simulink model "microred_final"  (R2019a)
settings: Solver=VariableStepAuto  StartTime=0.0  StopTime=24*60*60  FixedStep=1  RelTol=1e-3
undefined symbols (not defined in the file): A, B, C, cargagenerador, CoeficienteProduccion, Consumo_valores, consumogenerador, D1, Dd, Delta, irradiancia_valores, j, magnitude, PotenciaAerogenerador, precioelectricidad_valores, Precioventaelectricidad, Tiempo, VelocidadAerogenerador, viento_valores
libraries: powerlib x42, powerlib_meascontrol x6
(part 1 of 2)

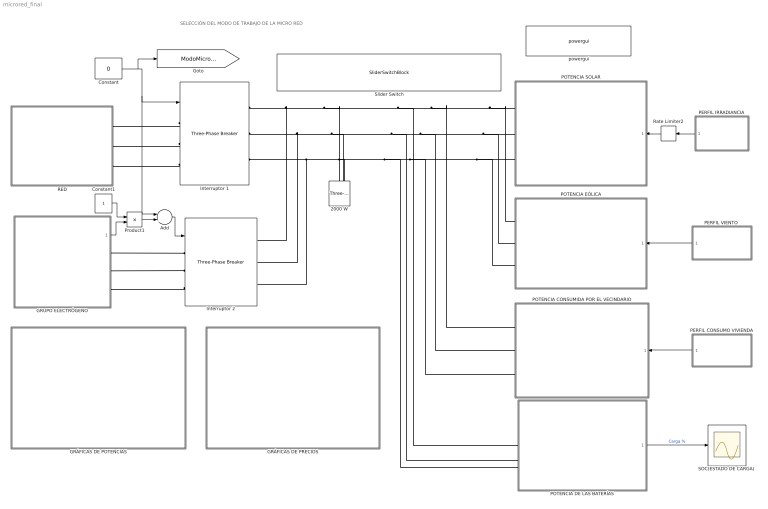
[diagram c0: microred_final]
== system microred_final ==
  note: SELECCIÓN DEL MODO DE TRABAJO DE LA MICRO RED
  2000 W : powerlib/Elements/Three-Phase Series RLC Load  LConnTagsString=A|B|C  Configuration=Y (grounded)  NominalVoltage=25e3  Vabc=[1e3 1e3 1e3]  Vabcp=[1e3 1e3 1e3]  NominalFrequency=50  UnbalancedPower=off  ActivePower=2000  InductivePower=0  CapacitivePower=0  Pabc=[10e3 9e3 11e3]  QLabc=[100 90 110]  QCabc=[100 90 110]  Pabcp=[10e3 9e3 11e3]  QLabcp=[100 90 110]  QCabcp=[100 90 110]  Measurements=None  LoadType=constant Z
  Add : Sum  Inputs=-+
  Constant : Constant  Value=0
  Constant1 : Constant
  GRUPO ELECTRÓGENO : Subsystem  mask{Voltaje=380, PotenciaMax=400}
      mask prompts: Voltaje "Voltaje (v)"; PotenciaMax "Potencia máxima (KW)"
  GRÁFICAS DE POTENCIAS : Subsystem
  GRÁFICAS DE PRECIOS : Subsystem
  Interruptor 1 : powerlib/Elements/Three-Phase Breaker  InitialState=closed  SwitchA=on  SwitchB=on  SwitchC=on  SwitchTimes="[1/60  5/60]"  External=on  BreakerResistance=0.001  SnubberResistance=100e6  SnubberCapacitance=0  Measurements=None
  Interruptor 2 : powerlib/Elements/Three-Phase Breaker  InitialState=closed  SwitchA=on  SwitchB=on  SwitchC=on  SwitchTimes="[1/60  5/60]"  External=on  BreakerResistance=0.001  SnubberResistance=inf  SnubberCapacitance=0  Measurements=None
  PERFIL CONSUMO VIVIENDA : Subsystem
      mask init:
      | load microred
  PERFIL IRRADIANCIA : Subsystem
      mask init:
      | load microred
  "PERFIL VIENTO " : Subsystem
      mask init:
      | load microred
  POTENCIA CONSUMIDA POR EL VECINDARIO : Subsystem  mask{NumCasas=1200, Fdp=0.8}
      mask prompts: NumCasas "Número de Casas"; Fdp "Factor de Potencia(0.8-1)"
  POTENCIA DE LAS BATERÍAS : Subsystem  mask{Rendimiento=95, Capacidad=4600, Vbat=400, Pbat=9200, NumBat=200, L_Sup=85, L_Inf=15, EstadoInicial=49.400, ModoEnergetico=Optimización de la energia}
      mask prompts: Rendimiento "Rendimiento de las baterías(%)"; Capacidad "Capacidad de las baterías(Ah)"; Vbat "Tensión de las baterías"; Pbat "Potencia de cada batería"; NumBat "Número de baterías"; L_Sup "Limite supeior SOC baterías"; L_Inf "Limite infeior SOC baterías"; EstadoInicial "Estado Inicial De la Carga(%)"; ModoEnergetico "Modo concetado a red"
  POTENCIA EÓLICA : Subsystem  mask{Modo=Curva de potencia, Densidad=1.225, SupViento=75.4, NumAerogeneradores=20, Fp=0.95}
      mask prompts: Modo "Modo de trabajo"; Densidad "Densidad del viento (kg/m^3)"; SupViento "Superficie de viento que incide en las aspas (m2)"; NumAerogeneradores "Número de aerogeneradores"; Fp "Factor de potencia ( 0.9-1)"
  POTENCIA SOLAR : Subsystem  mask{AreaPanel=1.77, NumPaneles=600, RendimientoPanel=22.6, Fdp=0.95}
      mask prompts: AreaPanel "Área de Cada Panel Solar (m^2)"; NumPaneles "Número de Paneles Solares"; RendimientoPanel "Rendimiento de los paneles solares (%)"; Fdp "Factor de Potencia (0.9-1)"
  Product1 : Product
  RED : Subsystem
  Rate Limiter2 : RateLimiter  RisingSlewLimit=1e7  FallingSlewLimit=-1e7  SampleTimeMode=inherited
  "SOC(ESTADO DE CARGA) " : Scope
  Slider Switch : SliderSwitchBlock
  powergui : powerlib/powergui  Priority=1  SimulationMode=Phasor  SampleTime=50e-6  frequency=50  Iterations=50  frequencyindice=50  Pbase=100e6  ErrMax=1e-4  UnitsV=kV  UnitsW=MW  buscounter=0  FunctionMessages=off  echomessages=off  EnableUseOfTLC=off  CurrentSourceSwitches=off  DisableSnubberDevices=off  DisableRonSwitches=off  DisableVfSwitches=off  DisplayEquations=off  AutomaticDiscreteSolvers=off  SolverType=Tustin/Backward Euler (TBE)  Interpol=off  ExternalGateDelay=off  methode=off  Ts=100  x0status=blocks  SPID=on  SwTol=0  HookPort=off  NonlinearTolerance=0  nMaxIteration=15  ContinueOnMaxIteration=off  RestoreLinks=warning  ResistiveCurrentMeasurement=off  Frange=[0:2:500]  Ylog=off  Xlog=on  ShowGrid=off  save=off  variable=ZData  structure=0  ZoomFFT=off  StartTime=0.0  cycles=1  DisplayStyle=1  fundamental=60  FreqAxis=off  MaxFrequency=1000  frequencyindicesteady=1  RmsSteady=1  display=off
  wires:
  POTENCIA DE LAS BATERÍAS/1(SOC) -> "SOC(ESTADO DE CARGA) "/1  "Carga %"
  Constant1/1 -> Product1/1
  GRUPO ELECTRÓGENO/1(Valor Coparacion Potencias) -> Product1/2
  Add/1 -> Interruptor 2/1
  Product1/1 -> Add/2
  Rate Limiter2/1 -> POTENCIA SOLAR/1(Perfil irradiancia)
  PERFIL CONSUMO VIVIENDA/1(Out2) -> POTENCIA CONSUMIDA POR EL VECINDARIO/1("Perfil consumo vivienda ")
  "PERFIL VIENTO "/1(Out2) -> POTENCIA EÓLICA/1(Perfil de viento)
  PERFIL IRRADIANCIA/1(Out1) -> Rate Limiter2/1
  Constant/1 -> [ModoMicrorred], Add/1, Interruptor 1/1
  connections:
  Interruptor 1/RConn2 -- Interruptor 2/RConn2 -- POTENCIA EÓLICA/RConn2 -- POTENCIA SOLAR/RConn2 -- POTENCIA CONSUMIDA POR EL VECINDARIO/RConn2 -- POTENCIA DE LAS BATERÍAS/LConn2 -- 2000 W/LConn2
  Interruptor 1/RConn3 -- Interruptor 2/RConn3 -- POTENCIA CONSUMIDA POR EL VECINDARIO/RConn3 -- POTENCIA EÓLICA/RConn3 -- POTENCIA SOLAR/RConn3 -- POTENCIA DE LAS BATERÍAS/LConn3 -- 2000 W/LConn3
  Interruptor 1/RConn1 -- Interruptor 2/RConn1 -- POTENCIA SOLAR/RConn1 -- POTENCIA EÓLICA/RConn1 -- POTENCIA CONSUMIDA POR EL VECINDARIO/RConn1 -- POTENCIA DE LAS BATERÍAS/LConn1 -- 2000 W/LConn1
  Interruptor 2/LConn3 -- GRUPO ELECTRÓGENO/RConn3
  Interruptor 2/LConn1 -- GRUPO ELECTRÓGENO/RConn1
  Interruptor 1/LConn3 -- RED/RConn3
  Interruptor 2/LConn2 -- GRUPO ELECTRÓGENO/RConn2
  Interruptor 1/LConn2 -- RED/RConn2
  Interruptor 1/LConn1 -- RED/RConn1

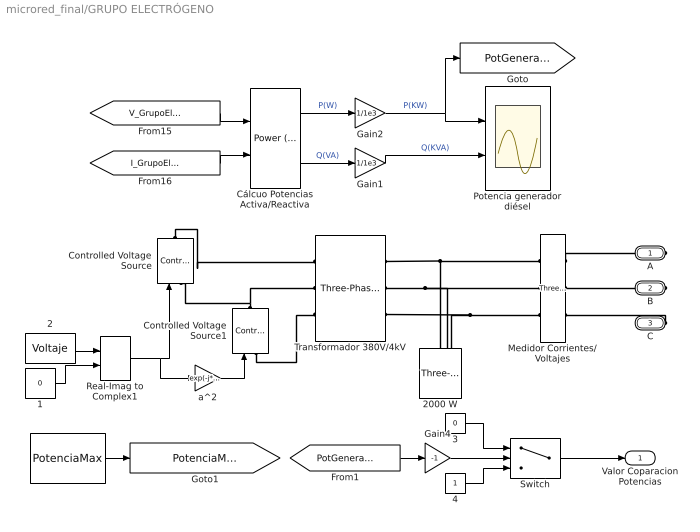
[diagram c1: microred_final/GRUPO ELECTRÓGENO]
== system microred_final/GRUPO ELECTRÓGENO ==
  " " : Constant  Value=PotenciaMax
  1 : Constant  Value=0
  2 : Constant  Value=Voltaje
  2000 W : powerlib/Elements/Three-Phase Series RLC Load  LConnTagsString=A|B|C  Configuration=Y (grounded)  NominalVoltage=25e3  Vabc=[1e3 1e3 1e3]  Vabcp=[1e3 1e3 1e3]  NominalFrequency=50  UnbalancedPower=off  ActivePower=2000  InductivePower=0  CapacitivePower=0  Pabc=[10e3 9e3 11e3]  QLabc=[100 90 110]  QCabc=[100 90 110]  Pabcp=[10e3 9e3 11e3]  QLabcp=[100 90 110]  QCabcp=[100 90 110]  Measurements=None  LoadType=constant Z
  3 : Constant  Value=0
  4 : Constant
  Controlled Voltage Source : powerlib/Electrical Sources/Controlled Voltage Source  Initialize=on  Source_Type=AC  Amplitude=0  Phase=0  Frequency=50  Measurements=None
  Controlled Voltage Source1 : powerlib/Electrical Sources/Controlled Voltage Source  Initialize=on  Source_Type=AC  Amplitude=0  Phase=0  Frequency=50  Measurements=None
  Cálcuo Potencias Activa/Reactiva : powerlib_meascontrol/Measurements/Power (3ph, Phasor)
  Gain1 : Gain  Gain=1/1e3
  Gain2 : Gain  Gain=1/1e3
  Gain4 : Gain  Gain=-1
  Medidor Corrientes/Voltajes : powerlib/Measurements/Three-Phase V-I Measurement  VoltageMeasurement=phase-to-ground  SetLabelV=on  LabelV=V_GrupoElectrogeno  Vpu=off  VpuLL=off  CurrentMeasurement=yes  SetLabelI=on  LabelI=I_GrupoElectrogeno  Ipu=off  Pbase=2*1.5e6/0.9  Vbase=25e3  OutputType=Complex  PhasorSimulation=on  PSBequivalent=0
  Potencia generador diésel : Scope  NumInputPorts=2
  Real-Imag to Complex1 : RealImagToComplex
  Switch : Switch  Criteria=u2 > Threshold  Threshold=PotenciaMax
  Transformador 380V/4kV : powerlib/Elements/Three-Phase Transformer (Two Windings)  Winding1Connection=Delta (D1)  Winding2Connection=Yg  CoreType=Three single-phase transformers  SetSaturation=off  Hysteresis=off  DataFile='hysteresis'  SetInitialFlux=off  Measurements=None  UNITS=pu  NominalPower=[ 20e6 , 60 ]  Winding1=[Voltaje, 0.002 , 0.08 ]  Winding2=[ 4000 , 0.002 , 0.08 ]  Rm=500  Lm=500  L0=0.5  Saturation=[ 0,0 ; 0.0024,1.2 ; 1.0,1.52 ]  InitialFluxes=[ 0.8 , -0.8 , 0.7 ]  BreakLoop=off  DiscreteSolver=Trapezoidal iterative  DataType=off  TransfoNumber=1
  a^2 : Gain  Gain=exp(-j*2*pi/3)
  A : PMIOPort  Side=Right
  B : PMIOPort  Port=2  Side=Right
  C : PMIOPort  Port=3  Side=Right
  Valor Coparacion Potencias : Outport
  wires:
  2/1 -> Real-Imag to Complex1/1
  Cálcuo Potencias Activa/Reactiva/2 -> Gain1/1  "Q(VA)"
  Gain1/1 -> Potencia generador diésel/2  "Q(KVA)"
  [V_GrupoElectrogeno] -> Cálcuo Potencias Activa/Reactiva/1
  Cálcuo Potencias Activa/Reactiva/1 -> Gain2/1  "P(W)"
  Gain2/1 -> Potencia generador diésel/1, [PotGeneradorDiesel]  "P(KW)"
  1/1 -> Real-Imag to Complex1/2
  Real-Imag to Complex1/1 -> a^2/1, Controlled Voltage Source/1
  [I_GrupoElectrogeno] -> Cálcuo Potencias Activa/Reactiva/2
  a^2/1 -> Controlled Voltage Source1/1
  4/1 -> Switch/3
  3/1 -> Switch/1
  Switch/1 -> Valor Coparacion Potencias/1
  [PotGeneradorDiesel] -> Gain4/1
  Gain4/1 -> Switch/2
  " "/1 -> [PotenciaMaximaGenerador]
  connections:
  Controlled Voltage Source1/RConn1 -- Controlled Voltage Source/LConn1 -- Transformador 380V/4kV/LConn2
  B/RConn1 -- Medidor Corrientes/Voltajes/RConn2
  Medidor Corrientes/Voltajes/RConn1 -- A/RConn1
  Controlled Voltage Source/RConn1 -- Transformador 380V/4kV/LConn1
  Controlled Voltage Source1/LConn1 -- Transformador 380V/4kV/LConn3
  C/RConn1 -- Medidor Corrientes/Voltajes/RConn3
  Medidor Corrientes/Voltajes/LConn1 -- Transformador 380V/4kV/RConn1 -- 2000 W/LConn1
  Transformador 380V/4kV/RConn2 -- 2000 W/LConn2 -- Medidor Corrientes/Voltajes/LConn2
  Medidor Corrientes/Voltajes/LConn3 -- Transformador 380V/4kV/RConn3 -- 2000 W/LConn3

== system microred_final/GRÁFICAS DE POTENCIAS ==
  note: Potencias Renovables
  note: Potencias Totales
  Add : Sum
  Gain : Gain  Gain=-1
  Potencias Renovables : Scope  NumInputPorts=3
  Potencias Totales : Scope  NumInputPorts=6
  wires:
  [PotEolica] -> Potencias Totales/2  "Eólica(azul)"
  [PotSolar] -> Potencias Totales/1  "Solar(rojo)"
  [Pbat] -> Potencias Totales/4  "Baterias(amarillo)"
  [PotGeneradorDiesel] -> Potencias Totales/6  "Diesel(marrón)"
  [PotRed] -> Potencias Totales/5  "Red(verde)"
  [PotSolar] -> Potencias Renovables/1, Add/1  "Solar"
  [PotEolica] -> Add/2, Potencias Renovables/2  "Eólica"
  Add/1 -> Potencias Renovables/3  "Potencia Renovables"
  Gain/1 -> Potencias Totales/3  "Consumida(morado)"
  [PotConsumida] -> Gain/1

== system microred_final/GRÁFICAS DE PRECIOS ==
  note: Precios micro red modo isla
  note: Precios micro red modo concetado a red
  Add2 : Sum  Inputs=+-
  Cálculo Precio Compra Electricidad : Subsystem
      mask init:
      | load microred
  Cálculo Precio Diesel : Subsystem
      mask init:
      | load microred
  Cálculo Precio Venta Electricidad : Subsystem
      mask init:
      | load microred
  Precio Diesel : Scope
  Precio total compra : Display
  Precio total de la micro red : Display
  Precio total diesel : Display
  Precio total venta : Display
  Precios Compra/venta : Scope  NumInputPorts=2
  Precios totales de la micro red : Scope
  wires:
  Cálculo Precio Compra Electricidad/1("Precio compra electricidad ") -> Add2/1, Precio total compra/1, Precios Compra/venta/1
  Cálculo Precio Venta Electricidad/1(Precio venta electricidad) -> Add2/2, Precio total venta/1, Precios Compra/venta/2
  Cálculo Precio Diesel/1(Precio Diesel) -> Precio total diesel/1, Precio Diesel/1
  Add2/1 -> Precio total de la micro red/1, Precios totales de la micro red/1

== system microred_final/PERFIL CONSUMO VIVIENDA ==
  note: Tabla Consumo Viviendas
  note: Segundos-->Horas
  1-D Lookup Table : Lookup_n-D  NumberOfTableDimensions=1  BreakpointsForDimension1=Tiempo  Table=Consumo_valores  InternalRulePriority=Speed  RndMeth=Simplest
  Clock : Clock
  Consumo : Scope
  Gain : Gain  Gain=1/(60*60)
  Out2 : Outport  VectorParamsAs1DForOutWhenUnconnected=on
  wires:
  Clock/1 -> Gain/1
  Gain/1 -> 1-D Lookup Table/1
  1-D Lookup Table/1 -> Out2/1, Consumo/1

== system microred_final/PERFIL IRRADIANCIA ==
  note: Tabla de Irradiancia
  note: Segundos-->Horas
  1-D Lookup Table : Lookup_n-D  NumberOfTableDimensions=1  BreakpointsForDimension1=Tiempo  Table=irradiancia_valores  InternalRulePriority=Speed  RndMeth=Simplest
  Clock : Clock
  Gain : Gain  Gain=1/(60*60)
  Irradiancia : Scope
  Scope1 : Scope
  Scope2 : Scope
  Out1 : Outport  VectorParamsAs1DForOutWhenUnconnected=on
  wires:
  Clock/1 -> Scope2/1, Gain/1
  Gain/1 -> Scope1/1, 1-D Lookup Table/1
  1-D Lookup Table/1 -> Irradiancia/1, Out1/1

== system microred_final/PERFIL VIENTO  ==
  note: Tabla de la velocidad del viento
  note: Segundos-->Horas
  1-D Lookup Table : Lookup_n-D  NumberOfTableDimensions=1  BreakpointsForDimension1=Tiempo  Table=viento_valores  InternalRulePriority=Speed  RndMeth=Simplest
  Clock : Clock
  Gain : Gain  Gain=1/(60*60)
  Viento : Scope
  Out2 : Outport  VectorParamsAs1DForOutWhenUnconnected=on
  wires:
  1-D Lookup Table/1 -> Out2/1, Viento/1
  Clock/1 -> Gain/1
  Gain/1 -> 1-D Lookup Table/1

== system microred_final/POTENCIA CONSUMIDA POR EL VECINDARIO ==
  "Perfil consumo vivienda " : Inport
  Cálclo potencia consumida por el vecindario : Subsystem
  Cálcuo Potencias Activa/Reactiva : powerlib_meascontrol/Measurements/Power (3ph, Phasor)
  Gain2 : Gain  Gain=1/1e3
  Gain3 : Gain  Gain=1/1e3
  Medidor Corrientes/Voltajes : powerlib/Measurements/Three-Phase V-I Measurement  VoltageMeasurement=phase-to-ground  SetLabelV=on  LabelV=Vconsumida  Vpu=off  VpuLL=off  CurrentMeasurement=yes  SetLabelI=on  LabelI=Iconsumida  Ipu=off  Pbase=100e6  Vbase=500e3  OutputType=Complex  PhasorSimulation=on  PSBequivalent=0
  Potencia consumida : Scope  NumInputPorts=2
  A : PMIOPort  Tag=PMCPort  Side=Right
  B : PMIOPort  Tag=PMCPort  Port=2  Side=Right
  C : PMIOPort  Tag=PMCPort  Port=3  Side=Right
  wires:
  "Perfil consumo vivienda "/1 -> Cálclo potencia consumida por el vecindario/1(Perfil de consumo)
  Cálcuo Potencias Activa/Reactiva/2 -> Gain2/1  "Q(VA)"
  [Iconsumida] -> Cálcuo Potencias Activa/Reactiva/2
  Gain3/1 -> Potencia consumida/1, [PotConsumida]  "P(KW)"
  [Vconsumida] -> Cálcuo Potencias Activa/Reactiva/1
  Gain2/1 -> Potencia consumida/2  "Q(KVA)"
  Cálcuo Potencias Activa/Reactiva/1 -> Gain3/1  "P(W)"
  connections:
  Medidor Corrientes/Voltajes/LConn1 -- Cálclo potencia consumida por el vecindario/RConn1
  Cálclo potencia consumida por el vecindario/RConn2 -- Medidor Corrientes/Voltajes/LConn2
  Cálclo potencia consumida por el vecindario/RConn3 -- Medidor Corrientes/Voltajes/LConn3
  Medidor Corrientes/Voltajes/RConn1 -- A/RConn1
  Medidor Corrientes/Voltajes/RConn2 -- B/RConn1
  Medidor Corrientes/Voltajes/RConn3 -- C/RConn1

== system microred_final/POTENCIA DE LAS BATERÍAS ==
  Cálculo potencia de las baterias : Subsystem
  Cálcuo Potencias Activa/Reactiva : powerlib_meascontrol/Measurements/Power (3ph, Phasor)
  Gain2 : Gain  Gain=1/1e3
  Gain3 : Gain  Gain=1/1e3
  "Medidor Corrientes/Voltajes " : powerlib/Measurements/Three-Phase V-I Measurement  VoltageMeasurement=phase-to-ground  SetLabelV=on  LabelV=Vbat  Vpu=off  VpuLL=off  CurrentMeasurement=yes  SetLabelI=on  LabelI=Ibat  Ipu=off  Pbase=100e6  Vbase=500e3  OutputType=Complex  PhasorSimulation=on  PSBequivalent=0
  Potencia Baterias : Scope  NumInputPorts=2
  A : PMIOPort  Tag=PMCPort  Side=Left
  B : PMIOPort  Tag=PMCPort  Port=2  Side=Left
  C : PMIOPort  Tag=PMCPort  Port=3  Side=Left
  SOC : Outport
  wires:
  Gain3/1 -> Potencia Baterias/1, [Pbat]  "P(KW)"
  [Vbat] -> Cálcuo Potencias Activa/Reactiva/1
  [Ibat] -> Cálcuo Potencias Activa/Reactiva/2
  Cálcuo Potencias Activa/Reactiva/2 -> Gain2/1  "Q(VA)"
  Gain2/1 -> Potencia Baterias/2  "Q(KVA)"
  Cálcuo Potencias Activa/Reactiva/1 -> Gain3/1  "P(W)"
  Cálculo potencia de las baterias/1(SOC) -> SOC/1
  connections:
  Cálculo potencia de las baterias/RConn1 -- "Medidor Corrientes/Voltajes "/LConn1
  "Medidor Corrientes/Voltajes "/LConn2 -- Cálculo potencia de las baterias/RConn2
  Cálculo potencia de las baterias/RConn3 -- "Medidor Corrientes/Voltajes "/LConn3
  "Medidor Corrientes/Voltajes "/RConn1 -- A/RConn1
  B/RConn1 -- "Medidor Corrientes/Voltajes "/RConn2
  "Medidor Corrientes/Voltajes "/RConn3 -- C/RConn1

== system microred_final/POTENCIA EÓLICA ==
  Perfil de viento : Inport
  Cálculo Potencias Activa/Reactiva : powerlib_meascontrol/Measurements/Power (3ph, Phasor)
  Cálculo potencia eólica : Subsystem
  Gain2 : Gain  Gain=1/1e3
  Gain3 : Gain  Gain=1/1e3
  Medidor Corrientes/Voltajes : powerlib/Measurements/Three-Phase V-I Measurement  VoltageMeasurement=phase-to-ground  SetLabelV=on  LabelV=Veolica  Vpu=off  VpuLL=off  CurrentMeasurement=yes  SetLabelI=on  LabelI=Ieolica  Ipu=off  Pbase=100e6  Vbase=500e3  OutputType=Complex  PhasorSimulation=on  PSBequivalent=0
  Potencia Eólica : Scope  NumInputPorts=2
  A : PMIOPort  Tag=PMCPort  Side=Right
  B : PMIOPort  Tag=PMCPort  Port=2  Side=Right
  C : PMIOPort  Tag=PMCPort  Port=3  Side=Right
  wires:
  Perfil de viento/1 -> Cálculo potencia eólica/1(Perfil de viento)
  Cálculo Potencias Activa/Reactiva/2 -> Gain2/1  "Q(VA)"
  [Ieolica] -> Cálculo Potencias Activa/Reactiva/2
  Gain3/1 -> Potencia Eólica/1, [PotEolica]  "P(KW)"
  [Veolica] -> Cálculo Potencias Activa/Reactiva/1
  Gain2/1 -> Potencia Eólica/2  "Q(KVA)"
  Cálculo Potencias Activa/Reactiva/1 -> Gain3/1  "P(W)"
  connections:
  Medidor Corrientes/Voltajes/RConn1 -- A/RConn1
  B/RConn1 -- Medidor Corrientes/Voltajes/RConn2
  C/RConn1 -- Medidor Corrientes/Voltajes/RConn3
  Medidor Corrientes/Voltajes/LConn3 -- Cálculo potencia eólica/RConn3
  Medidor Corrientes/Voltajes/LConn2 -- Cálculo potencia eólica/RConn2
  Medidor Corrientes/Voltajes/LConn1 -- Cálculo potencia eólica/RConn1

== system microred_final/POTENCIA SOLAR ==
  Perfil irradiancia : Inport
  "Cálculo potencia solar " : Subsystem
  Cálcuo Potencias Activa/Reactiva : powerlib_meascontrol/Measurements/Power (3ph, Phasor)
  Gain2 : Gain  Gain=1/1e3
  Gain3 : Gain  Gain=1/1e3
  Medidor Corrientes/Voltajes : powerlib/Measurements/Three-Phase V-I Measurement  VoltageMeasurement=phase-to-ground  SetLabelV=on  LabelV=Vsol  Vpu=off  VpuLL=off  CurrentMeasurement=yes  SetLabelI=on  LabelI=Isol  Ipu=off  Pbase=100e6  Vbase=500e3  OutputType=Complex  PhasorSimulation=on  PSBequivalent=0
  Potencia Solar : Scope  NumInputPorts=2
  A : PMIOPort  Tag=PMCPort  Side=Right
  B : PMIOPort  Tag=PMCPort  Port=2  Side=Right
  C : PMIOPort  Tag=PMCPort  Port=3  Side=Right
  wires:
  Perfil irradiancia/1 -> "Cálculo potencia solar "/1(Perfil de irradiancia)
  Cálcuo Potencias Activa/Reactiva/1 -> Gain3/1  "P(W)"
  [Isol] -> Cálcuo Potencias Activa/Reactiva/2
  [Vsol] -> Cálcuo Potencias Activa/Reactiva/1
  Cálcuo Potencias Activa/Reactiva/2 -> Gain2/1  "Q(VA)"
  Gain2/1 -> Potencia Solar/2  "Q(KVA)"
  Gain3/1 -> [PotSolar], Potencia Solar/1  "P(KW)"
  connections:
  "Cálculo potencia solar "/RConn1 -- Medidor Corrientes/Voltajes/LConn1
  "Cálculo potencia solar "/RConn2 -- Medidor Corrientes/Voltajes/LConn2
  "Cálculo potencia solar "/RConn3 -- Medidor Corrientes/Voltajes/LConn3
  Medidor Corrientes/Voltajes/RConn1 -- A/RConn1
  Medidor Corrientes/Voltajes/RConn2 -- B/RConn1
  C/RConn1 -- Medidor Corrientes/Voltajes/RConn3

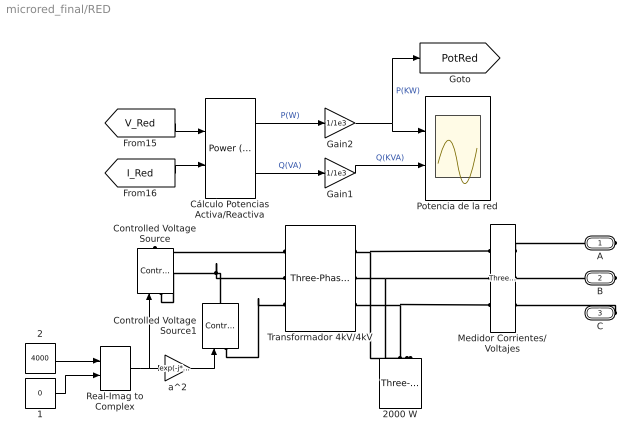
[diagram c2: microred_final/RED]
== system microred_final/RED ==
  1 : Constant  Value=0
  2 : Constant  Value=4000
  2000 W : powerlib/Elements/Three-Phase Series RLC Load  LConnTagsString=A|B|C  Configuration=Y (grounded)  NominalVoltage=25e3  Vabc=[1e3 1e3 1e3]  Vabcp=[1e3 1e3 1e3]  NominalFrequency=50  UnbalancedPower=off  ActivePower=2000  InductivePower=0  CapacitivePower=0  Pabc=[10e3 9e3 11e3]  QLabc=[100 90 110]  QCabc=[100 90 110]  Pabcp=[10e3 9e3 11e3]  QLabcp=[100 90 110]  QCabcp=[100 90 110]  Measurements=None  LoadType=constant Z
  Controlled Voltage Source : powerlib/Electrical Sources/Controlled Voltage Source  Initialize=on  Source_Type=AC  Amplitude=0  Phase=0  Frequency=50  Measurements=None
  Controlled Voltage Source1 : powerlib/Electrical Sources/Controlled Voltage Source  Initialize=on  Source_Type=AC  Amplitude=0  Phase=0  Frequency=50  Measurements=None
  Cálculo Potencias Activa/Reactiva : powerlib_meascontrol/Measurements/Power (3ph, Phasor)
  Gain1 : Gain  Gain=1/1e3
  Gain2 : Gain  Gain=1/1e3
  Medidor Corrientes/Voltajes : powerlib/Measurements/Three-Phase V-I Measurement  VoltageMeasurement=phase-to-ground  SetLabelV=on  LabelV=V_Red  Vpu=off  VpuLL=off  CurrentMeasurement=yes  SetLabelI=on  LabelI=I_Red  Ipu=off  Pbase=2*1.5e6/0.9  Vbase=25e3  OutputType=Complex  PhasorSimulation=on  PSBequivalent=0
  Potencia de la red : Scope  NumInputPorts=2
  Real-Imag to Complex : RealImagToComplex
  Transformador 4kV/4kV : powerlib/Elements/Three-Phase Transformer (Two Windings)  Winding1Connection=Delta (D1)  Winding2Connection=Yg  CoreType=Three single-phase transformers  SetSaturation=off  Hysteresis=off  DataFile='hysteresis'  SetInitialFlux=off  Measurements=None  UNITS=pu  NominalPower=[ 20e6 , 60 ]  Winding1=[4000 , 0.002 , 0.08 ]  Winding2=[ 4000, 0.002 , 0.08 ]  Rm=500  Lm=500  L0=0.5  Saturation=[ 0,0 ; 0.0024,1.2 ; 1.0,1.52 ]  InitialFluxes=[ 0.8 , -0.8 , 0.7 ]  BreakLoop=off  DiscreteSolver=Trapezoidal iterative  DataType=off  TransfoNumber=1
  a^2 : Gain  Gain=exp(-j*2*pi/3)
  A : PMIOPort  Side=Right
  B : PMIOPort  Port=2  Side=Right
  C : PMIOPort  Port=3  Side=Right
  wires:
  Gain2/1 -> [PotRed], Potencia de la red/1  "P(KW)"
  Cálculo Potencias Activa/Reactiva/1 -> Gain2/1  "P(W)"
  [V_Red] -> Cálculo Potencias Activa/Reactiva/1
  [I_Red] -> Cálculo Potencias Activa/Reactiva/2
  Cálculo Potencias Activa/Reactiva/2 -> Gain1/1  "Q(VA)"
  Gain1/1 -> Potencia de la red/2  "Q(KVA)"
  a^2/1 -> Controlled Voltage Source1/1
  Real-Imag to Complex/1 -> Controlled Voltage Source/1, a^2/1
  2/1 -> Real-Imag to Complex/1
  1/1 -> Real-Imag to Complex/2
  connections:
  Medidor Corrientes/Voltajes/RConn1 -- A/RConn1
  C/RConn1 -- Medidor Corrientes/Voltajes/RConn3
  B/RConn1 -- Medidor Corrientes/Voltajes/RConn2
  Transformador 4kV/4kV/RConn2 -- Medidor Corrientes/Voltajes/LConn2 -- 2000 W/LConn2
  Transformador 4kV/4kV/RConn3 -- Medidor Corrientes/Voltajes/LConn3 -- 2000 W/LConn3
  Transformador 4kV/4kV/RConn1 -- Medidor Corrientes/Voltajes/LConn1 -- 2000 W/LConn1
  Controlled Voltage Source/RConn1 -- Transformador 4kV/4kV/LConn1
  Controlled Voltage Source/LConn1 -- Controlled Voltage Source1/RConn1 -- Transformador 4kV/4kV/LConn2
  Controlled Voltage Source1/LConn1 -- Transformador 4kV/4kV/LConn3

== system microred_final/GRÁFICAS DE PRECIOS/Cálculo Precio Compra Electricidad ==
  " " : Constant  Value=0
  Add1 : Sum
  Gain4 : Gain  Gain=1/(3600)
  "Perfil Precio Electricidad Compra " : Subsystem
      mask init:
      | load microred
  Precio Compra : Scope
  Product : Product
  Switch : Switch  Criteria=u2 > Threshold
  real1 : Subsystem  mask(Transfer Function with Initial Outputs){N=[1], D=[1 1], Y0=0, U0=0}
      mask prompts: N "Numerator:"; D "Denominator:"; Y0 "Initial output:"; U0 "Initial input:"
      mask help: Vector expressions for numerator, and denominator. Coefficients are in descending powers of s.
      mask init:
      | [A,B,C,Dd]=tf2ss(N,D);if (isempty(Y0));[m,n]=size(A);X0=zeros(1,m); end; if (isempty(U0));[m,p]=size(B);U0=zeros(1,p);end;X0=getxo(A,B,C,Dd,U0,Y0,0);
  "Precio compra electricidad " : Outport
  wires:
  Product/1 -> Gain4/1
  Gain4/1 -> Add1/1
  real1/1(Out1) -> Add1/2
  "Perfil Precio Electricidad Compra "/1(Out2) -> [PrecioCompra], Product/2
  " "/1 -> Switch/3
  Switch/1 -> Product/1
  [PotRed] -> Switch/1, Switch/2
  Add1/1 -> "Precio compra electricidad "/1, Precio Compra/1, real1/1(In1)

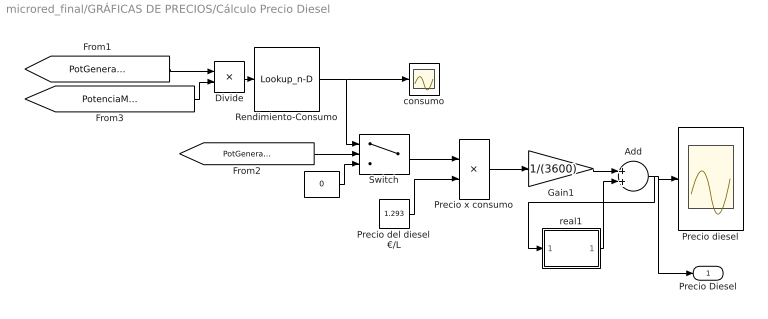
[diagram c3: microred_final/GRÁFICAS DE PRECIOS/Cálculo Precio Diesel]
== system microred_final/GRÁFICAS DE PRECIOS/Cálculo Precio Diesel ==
  " " : Constant  Value=0
  Add : Sum
  Divide : Product  Inputs=*/
  Gain1 : Gain  Gain=1/(3600)
  Precio del diesel €/L : Constant  Value=1.293
  Precio diesel : Scope
  Precio x consumo : Product
  Rendimiento-Consumo : Lookup_n-D  NumberOfTableDimensions=1  BreakpointsForDimension1=cargagenerador  Table=consumogenerador  InternalRulePriority=Speed  RndMeth=Simplest
  Switch : Switch  Criteria=u2 > Threshold
  consumo : Scope
  real1 : Subsystem  mask(Transfer Function with Initial Outputs){N=[1], D=[1 1], Y0=0, U0=0}
      mask prompts: N "Numerator:"; D "Denominator:"; Y0 "Initial output:"; U0 "Initial input:"
      mask help: Vector expressions for numerator, and denominator. Coefficients are in descending powers of s.
      mask init:
      | [A,B,C,Dd]=tf2ss(N,D);if (isempty(Y0));[m,n]=size(A);X0=zeros(1,m); end; if (isempty(U0));[m,p]=size(B);U0=zeros(1,p);end;X0=getxo(A,B,C,Dd,U0,Y0,0);
  Precio Diesel : Outport
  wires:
  Add/1 -> Precio Diesel/1, Precio diesel/1, real1/1(In1)
  real1/1(Out1) -> Add/2
  Precio del diesel €/L/1 -> Precio x consumo/2
  Switch/1 -> Precio x consumo/1
  [PotGeneradorDiesel] -> Divide/1
  Rendimiento-Consumo/1 -> Switch/1, consumo/1
  Divide/1 -> Rendimiento-Consumo/1
  [PotGeneradorDiesel] -> Switch/2
  " "/1 -> Switch/3
  [PotenciaMaximaGenerador] -> Divide/2
  Gain1/1 -> Add/1
  Precio x consumo/1 -> Gain1/1

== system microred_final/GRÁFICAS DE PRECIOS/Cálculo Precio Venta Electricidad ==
  " 1" : Constant  Value=0
  Add2 : Sum
  Gain1 : Gain  Gain=-1
  Gain2 : Gain  Gain=1/(3600)
  Gain3 : Gain  Gain=1e-3
  "Perfil Precio Electricidad Venta " : Subsystem
      mask init:
      | load microred
  Precio Venta : Scope
  Product1 : Product
  Switch : Switch  Criteria=u2 > Threshold
  real1 : Subsystem  mask(Transfer Function with Initial Outputs){N=[1], D=[1 1], Y0=0, U0=0}
      mask prompts: N "Numerator:"; D "Denominator:"; Y0 "Initial output:"; U0 "Initial input:"
      mask help: Vector expressions for numerator, and denominator. Coefficients are in descending powers of s.
      mask init:
      | [A,B,C,Dd]=tf2ss(N,D);if (isempty(Y0));[m,n]=size(A);X0=zeros(1,m); end; if (isempty(U0));[m,p]=size(B);U0=zeros(1,p);end;X0=getxo(A,B,C,Dd,U0,Y0,0);
  Precio venta electricidad : Outport
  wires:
  Product1/1 -> Gain2/1
  Gain2/1 -> Add2/1
  "Perfil Precio Electricidad Venta "/1(Out2) -> [PrecioVenta], Gain3/1
  real1/1(Out1) -> Add2/2
  Gain1/1 -> Product1/1
  [PotRed] -> Switch/3, Switch/2
  " 1"/1 -> Switch/1
  Switch/1 -> Gain1/1
  Add2/1 -> real1/1(In1), Precio Venta/1, Precio venta electricidad/1
  Gain3/1 -> Product1/2

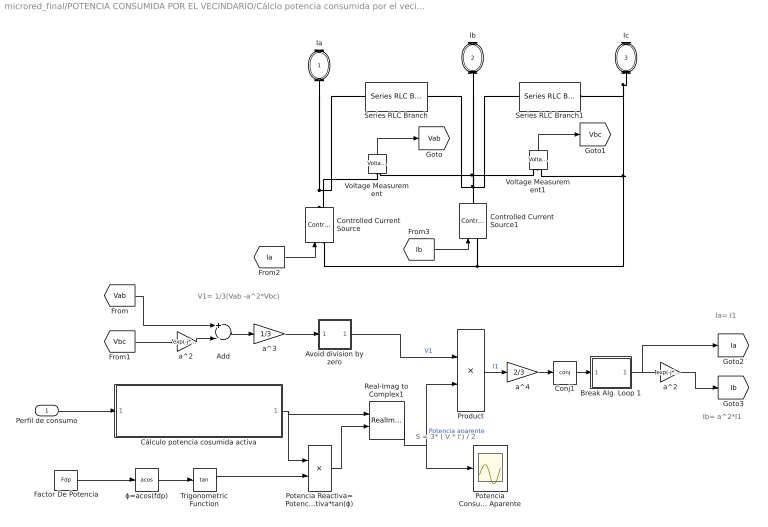
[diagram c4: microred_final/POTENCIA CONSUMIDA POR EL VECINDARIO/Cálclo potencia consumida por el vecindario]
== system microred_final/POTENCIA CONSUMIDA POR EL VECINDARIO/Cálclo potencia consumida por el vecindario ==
  note: V1= 1/3(Vab -a^2*Vbc)
  note: Ia= I1
  note: Ib= a^2*I1
  note: S = 3* ( V * I') / 2
  Perfil de consumo : Inport
  Add : Sum  Inputs=+-
  Avoid division by zero : Subsystem
  Break Alg. Loop 1 : Subsystem
  Conj1 : Math  Operator=conj
  Controlled Current Source : powerlib/Electrical Sources/Controlled Current Source  Initialize=on  Source_Type=AC  Amplitude=0  Phase=0  Frequency=50  Measurements=None
  Controlled Current Source1 : powerlib/Electrical Sources/Controlled Current Source  Initialize=on  Source_Type=AC  Amplitude=0  Phase=0  Frequency=50  Measurements=None
  Cálculo potencia cosumida activa : Subsystem
  Factor De Potencia : Constant  Value=Fdp
  Potencia Consumida Aparente : Scope
  Potencia Reactiva=Potencia Activa*tan(ϕ) : Product
  Product : Product  Inputs=/*
  Real-Imag to Complex1 : RealImagToComplex
  Series RLC Branch : powerlib/Elements/Series RLC Branch  LConnTagsString=__new0  RConnTagsString=__new0  BranchType=R  Resistance=1e6  Inductance=1e-3  SetiL0=off  InitialCurrent=0  Capacitance=1e-6  Setx0=off  InitialVoltage=0  Measurements=None
  Series RLC Branch1 : powerlib/Elements/Series RLC Branch  LConnTagsString=__new0  RConnTagsString=__new0  BranchType=R  Resistance=1e6  Inductance=1e-3  SetiL0=off  InitialCurrent=0  Capacitance=1e-6  Setx0=off  InitialVoltage=0  Measurements=None
  Trigonometric Function : Trigonometry  Operator=tan
  Voltage Measurement : powerlib/Measurements/Voltage Measurement  PhasorSimulation=on  OutputType=Complex  PSBequivalent=0
  Voltage Measurement1 : powerlib/Measurements/Voltage Measurement  PhasorSimulation=on  OutputType=Complex  PSBequivalent=0
  a^2 : Gain  Gain=exp(-j*2*pi/3)
  "a^2 " : Gain  Gain=exp(-j*2*pi/3)
  a^3 : Gain  Gain=1/3
  a^4 : Gain  Gain=2/3
  ϕ=acos(fdp) : Trigonometry  Operator=acos
  Ia : PMIOPort  Tag=PMCPort  Side=Right
  Ib : PMIOPort  Tag=PMCPort  Port=2  Side=Right
  Ic : PMIOPort  Tag=PMCPort  Port=3  Side=Right
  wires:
  Add/1 -> a^3/1
  "a^2 "/1 -> Add/2
  Product/1 -> a^4/1  "I1"
  a^4/1 -> Conj1/1
  Break Alg. Loop 1/1(Out) -> [Ia], a^2/1
  [Ia] -> Controlled Current Source/1
  Conj1/1 -> Break Alg. Loop 1/1(In)
  a^2/1 -> [Ib]
  Voltage Measurement/1 -> [Vab]
  Voltage Measurement1/1 -> [Vbc]
  [Ib] -> Controlled Current Source1/1
  [Vab] -> Add/1
  [Vbc] -> "a^2 "/1
  a^3/1 -> Avoid division by zero/1(I)
  Avoid division by zero/1(O) -> Product/1  "V1"
  Real-Imag to Complex1/1 -> Potencia Consumida Aparente/1, Product/2  "Potencia aparente"
  Factor De Potencia/1 -> ϕ=acos(fdp)/1
  ϕ=acos(fdp)/1 -> Trigonometric Function/1
  Trigonometric Function/1 -> Potencia Reactiva=Potencia Activa*tan(ϕ)/2
  Potencia Reactiva=Potencia Activa*tan(ϕ)/1 -> Real-Imag to Complex1/2
  Cálculo potencia cosumida activa/1(Potencia consumida activa) -> Real-Imag to Complex1/1, Potencia Reactiva=Potencia Activa*tan(ϕ)/1
  Perfil de consumo/1 -> Cálculo potencia cosumida activa/1(Perfil de consumo)
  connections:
  Controlled Current Source/LConn1 -- Controlled Current Source1/LConn1 -- Voltage Measurement1/LConn2 -- Series RLC Branch1/RConn1 -- Ic/RConn1
  Voltage Measurement/LConn1 -- Ia/RConn1 -- Series RLC Branch/LConn1 -- Controlled Current Source/RConn1
  Voltage Measurement/LConn2 -- Voltage Measurement1/LConn1 -- Series RLC Branch/RConn1 -- Ib/RConn1 -- Series RLC Branch1/LConn1 -- Controlled Current Source1/RConn1

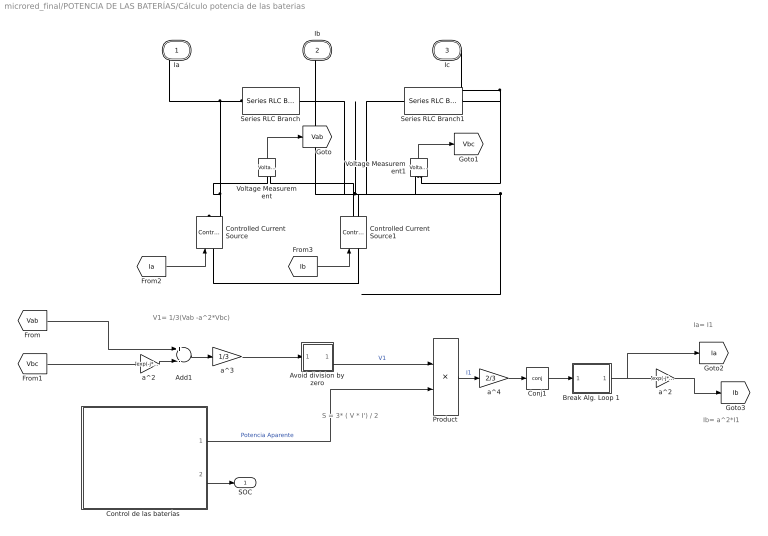
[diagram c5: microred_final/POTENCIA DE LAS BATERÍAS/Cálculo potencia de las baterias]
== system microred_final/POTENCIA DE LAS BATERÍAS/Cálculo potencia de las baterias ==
  note: Ia= I1
  note: V1= 1/3(Vab -a^2*Vbc)
  note: Ib= a^2*I1
  note: S = 3* ( V * I') / 2
  Add1 : Sum  Inputs=+-
  Avoid division by zero : Subsystem
  Break Alg. Loop 1 : Subsystem
  Conj1 : Math  Operator=conj
  "Control de las baterías " : Subsystem
  Controlled Current Source : powerlib/Electrical Sources/Controlled Current Source  Initialize=on  Source_Type=AC  Amplitude=0  Phase=0  Frequency=50  Measurements=None
  Controlled Current Source1 : powerlib/Electrical Sources/Controlled Current Source  Initialize=on  Source_Type=AC  Amplitude=0  Phase=0  Frequency=50  Measurements=None
  Product : Product  Inputs=/*
  Series RLC Branch : powerlib/Elements/Series RLC Branch  LConnTagsString=__new0  RConnTagsString=__new0  BranchType=R  Resistance=1e6  Inductance=1e-3  SetiL0=off  InitialCurrent=0  Capacitance=1e-6  Setx0=off  InitialVoltage=0  Measurements=None
  Series RLC Branch1 : powerlib/Elements/Series RLC Branch  LConnTagsString=__new0  RConnTagsString=__new0  BranchType=R  Resistance=1e6  Inductance=1e-3  SetiL0=off  InitialCurrent=0  Capacitance=1e-6  Setx0=off  InitialVoltage=0  Measurements=None
  Voltage Measurement : powerlib/Measurements/Voltage Measurement  PhasorSimulation=on  OutputType=Complex  PSBequivalent=0
  Voltage Measurement1 : powerlib/Measurements/Voltage Measurement  PhasorSimulation=on  OutputType=Complex  PSBequivalent=0
  a^2 : Gain  Gain=exp(-j*2*pi/3)
  "a^2 " : Gain  Gain=exp(-j*2*pi/3)
  a^3 : Gain  Gain=1/3
  a^4 : Gain  Gain=2/3
  Ia : PMIOPort  Tag=PMCPort  Side=Right
  Ib : PMIOPort  Tag=PMCPort  Port=2  Side=Right
  Ic : PMIOPort  Tag=PMCPort  Port=3  Side=Right
  SOC : Outport
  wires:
  Add1/1 -> a^3/1
  [Ia] -> Controlled Current Source/1
  a^3/1 -> Avoid division by zero/1(I)
  a^4/1 -> Conj1/1
  Break Alg. Loop 1/1(Out) -> [Ia], a^2/1
  "a^2 "/1 -> Add1/2
  Voltage Measurement/1 -> [Vab]
  Voltage Measurement1/1 -> [Vbc]
  Conj1/1 -> Break Alg. Loop 1/1(In)
  Product/1 -> a^4/1  "I1"
  [Ib] -> Controlled Current Source1/1
  a^2/1 -> [Ib]
  [Vbc] -> "a^2 "/1
  Avoid division by zero/1(O) -> Product/1  "V1"
  "Control de las baterías "/1(Potencia Baterías) -> Product/2  "Potencia Aparente"
  [Vab] -> Add1/1
  "Control de las baterías "/2(SOC) -> SOC/1
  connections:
  Voltage Measurement1/LConn2 -- Controlled Current Source/LConn1 -- Controlled Current Source1/LConn1 -- Ic/RConn1 -- Series RLC Branch1/RConn1
  Series RLC Branch/LConn1 -- Ia/RConn1 -- Voltage Measurement/LConn1 -- Controlled Current Source/RConn1
  Voltage Measurement1/LConn1 -- Voltage Measurement/LConn2 -- Controlled Current Source1/RConn1 -- Ib/RConn1 -- Series RLC Branch1/LConn1 -- Series RLC Branch/RConn1

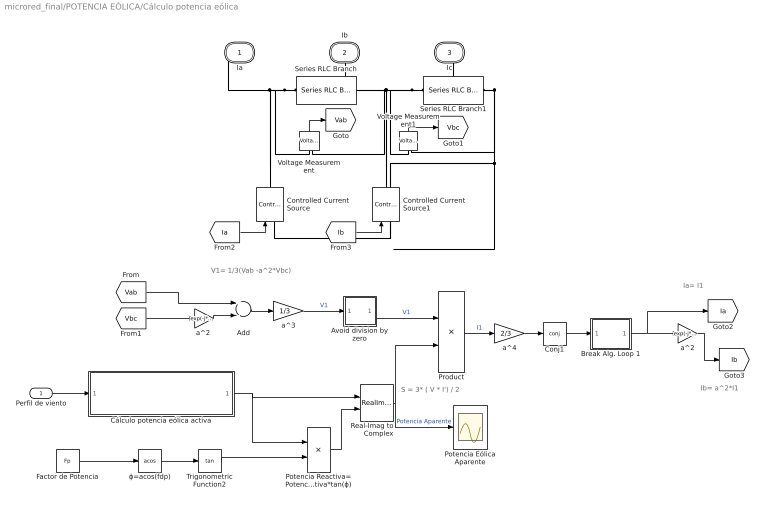
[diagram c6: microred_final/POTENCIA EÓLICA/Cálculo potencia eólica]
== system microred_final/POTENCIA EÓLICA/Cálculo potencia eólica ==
  note: Ia= I1
  note: V1= 1/3(Vab -a^2*Vbc)
  note: S = 3* ( V * I') / 2
  note: Ib= a^2*I1
  Perfil de viento : Inport
  Add : Sum  Inputs=+-
  Avoid division by zero : Subsystem
  Break Alg. Loop 1 : Subsystem
  Conj1 : Math  Operator=conj
  Controlled Current Source : powerlib/Electrical Sources/Controlled Current Source  Initialize=on  Source_Type=AC  Amplitude=0  Phase=0  Frequency=50  Measurements=None
  Controlled Current Source1 : powerlib/Electrical Sources/Controlled Current Source  Initialize=on  Source_Type=AC  Amplitude=0  Phase=0  Frequency=50  Measurements=None
  Cálculo potencia eólica activa : Subsystem
      mask init:
      | load microred
  Factor de Potencia : Constant  Value=Fp
  Potencia Eólica Aparente : Scope
  Potencia Reactiva=Potencia Activa*tan(ϕ) : Product
  Product : Product  Inputs=/*
  Real-Imag to Complex : RealImagToComplex
  Series RLC Branch : powerlib/Elements/Series RLC Branch  LConnTagsString=__new0  RConnTagsString=__new0  BranchType=R  Resistance=1e6  Inductance=1e-3  SetiL0=off  InitialCurrent=0  Capacitance=1e-6  Setx0=off  InitialVoltage=0  Measurements=None
  Series RLC Branch1 : powerlib/Elements/Series RLC Branch  LConnTagsString=__new0  RConnTagsString=__new0  BranchType=R  Resistance=1e6  Inductance=1e-3  SetiL0=off  InitialCurrent=0  Capacitance=1e-6  Setx0=off  InitialVoltage=0  Measurements=None
  Trigonometric Function2 : Trigonometry  Operator=tan
  Voltage Measurement : powerlib/Measurements/Voltage Measurement  PhasorSimulation=on  OutputType=Complex  PSBequivalent=0
  Voltage Measurement1 : powerlib/Measurements/Voltage Measurement  PhasorSimulation=on  OutputType=Complex  PSBequivalent=0
  a^2 : Gain  Gain=exp(-j*2*pi/3)
  "a^2 " : Gain  Gain=exp(-j*2*pi/3)
  a^3 : Gain  Gain=1/3
  a^4 : Gain  Gain=2/3
  ϕ=acos(fdp) : Trigonometry  Operator=acos
  Ia : PMIOPort  Tag=PMCPort  Side=Right
  Ib : PMIOPort  Tag=PMCPort  Port=2  Side=Right
  Ic : PMIOPort  Tag=PMCPort  Port=3  Side=Right
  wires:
  Real-Imag to Complex/1 -> Potencia Eólica Aparente/1, Product/2  "Potencia Aparente"
  Potencia Reactiva=Potencia Activa*tan(ϕ)/1 -> Real-Imag to Complex/2
  Add/1 -> a^3/1
  Conj1/1 -> Break Alg. Loop 1/1(In)
  Avoid division by zero/1(O) -> Product/1  "V1"
  Product/1 -> a^4/1  "I1"
  a^2/1 -> [Ib]
  [Vbc] -> "a^2 "/1
  Break Alg. Loop 1/1(Out) -> a^2/1, [Ia]
  "a^2 "/1 -> Add/2
  [Ia] -> Controlled Current Source/1
  a^4/1 -> Conj1/1
  [Ib] -> Controlled Current Source1/1
  [Vab] -> Add/1
  a^3/1 -> Avoid division by zero/1(I)  "V1"
  Voltage Measurement/1 -> [Vab]
  Voltage Measurement1/1 -> [Vbc]
  Cálculo potencia eólica activa/1(Potencia eólica activa) -> Real-Imag to Complex/1, Potencia Reactiva=Potencia Activa*tan(ϕ)/1
  Perfil de viento/1 -> Cálculo potencia eólica activa/1(Perfil de viento)
  ϕ=acos(fdp)/1 -> Trigonometric Function2/1
  Trigonometric Function2/1 -> Potencia Reactiva=Potencia Activa*tan(ϕ)/2
  Factor de Potencia/1 -> ϕ=acos(fdp)/1
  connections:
  Series RLC Branch1/RConn1 -- Controlled Current Source1/LConn1 -- Controlled Current Source/LConn1 -- Voltage Measurement1/LConn2 -- Ic/RConn1
  Series RLC Branch1/LConn1 -- Series RLC Branch/RConn1 -- Voltage Measurement1/LConn1 -- Voltage Measurement/LConn2 -- Controlled Current Source1/RConn1 -- Ib/RConn1
  Series RLC Branch/LConn1 -- Ia/RConn1 -- Controlled Current Source/RConn1 -- Voltage Measurement/LConn1

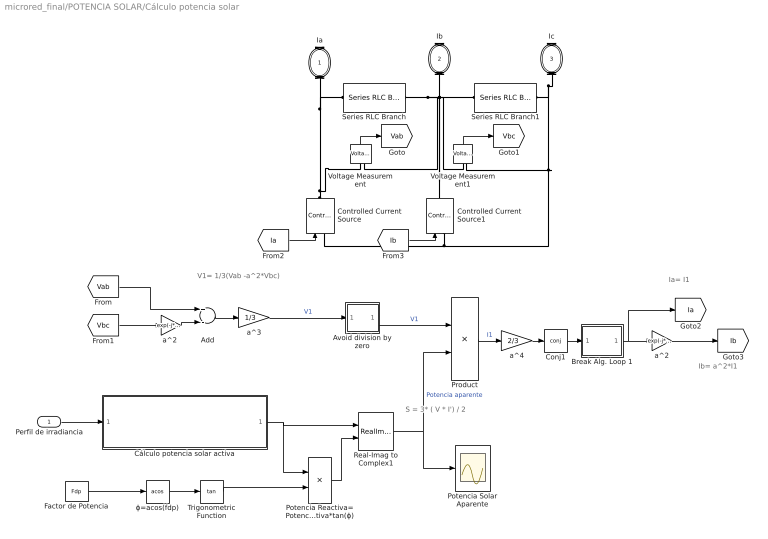
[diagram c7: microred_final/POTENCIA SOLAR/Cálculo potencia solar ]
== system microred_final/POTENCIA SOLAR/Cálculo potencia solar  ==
  note: Ia= I1
  note: V1= 1/3(Vab -a^2*Vbc)
  note: Ib= a^2*I1
  note: S = 3* ( V * I') / 2
  Perfil de irradiancia : Inport
  Add : Sum  Inputs=+-
  Avoid division by zero : Subsystem
  Break Alg. Loop 1 : Subsystem
  Conj1 : Math  Operator=conj
  Controlled Current Source : powerlib/Electrical Sources/Controlled Current Source  Initialize=on  Source_Type=AC  Amplitude=0  Phase=0  Frequency=50  Measurements=None
  Controlled Current Source1 : powerlib/Electrical Sources/Controlled Current Source  Initialize=on  Source_Type=AC  Amplitude=0  Phase=0  Frequency=50  Measurements=None
  Cálculo potencia solar activa : Subsystem
  Factor de Potencia : Constant  Value=Fdp
  Potencia Reactiva=Potencia Activa*tan(ϕ) : Product
  Potencia Solar Aparente : Scope
  Product : Product  Inputs=/*
  Real-Imag to Complex1 : RealImagToComplex
  Series RLC Branch : powerlib/Elements/Series RLC Branch  LConnTagsString=__new0  RConnTagsString=__new0  BranchType=R  Resistance=1e6  Inductance=1e-3  SetiL0=off  InitialCurrent=0  Capacitance=1e-6  Setx0=off  InitialVoltage=0  Measurements=None
  Series RLC Branch1 : powerlib/Elements/Series RLC Branch  LConnTagsString=__new0  RConnTagsString=__new0  BranchType=R  Resistance=1e6  Inductance=1e-3  SetiL0=off  InitialCurrent=0  Capacitance=1e-6  Setx0=off  InitialVoltage=0  Measurements=None
  Trigonometric Function : Trigonometry  Operator=tan
  Voltage Measurement : powerlib/Measurements/Voltage Measurement  PhasorSimulation=on  OutputType=Complex  PSBequivalent=0
  Voltage Measurement1 : powerlib/Measurements/Voltage Measurement  PhasorSimulation=on  OutputType=Complex  PSBequivalent=0
  a^2 : Gain  Gain=exp(-j*2*pi/3)
  "a^2 " : Gain  Gain=exp(-j*2*pi/3)
  a^3 : Gain  Gain=1/3
  a^4 : Gain  Gain=2/3
  ϕ=acos(fdp) : Trigonometry  Operator=acos
  Ia : PMIOPort  Tag=PMCPort  Side=Right
  Ib : PMIOPort  Tag=PMCPort  Port=2  Side=Right
  Ic : PMIOPort  Tag=PMCPort  Port=3  Side=Right
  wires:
  [Vab] -> Add/1
  [Ia] -> Controlled Current Source/1
  a^2/1 -> [Ib]
  Real-Imag to Complex1/1 -> Potencia Solar Aparente/1, Product/2  "Potencia aparente"
  [Vbc] -> "a^2 "/1
  Conj1/1 -> Break Alg. Loop 1/1(In)
  Break Alg. Loop 1/1(Out) -> [Ia], a^2/1
  [Ib] -> Controlled Current Source1/1
  a^4/1 -> Conj1/1
  "a^2 "/1 -> Add/2
  Product/1 -> a^4/1  "I1"
  Add/1 -> a^3/1
  Avoid division by zero/1(O) -> Product/1  "V1"
  a^3/1 -> Avoid division by zero/1(I)  "V1"
  Voltage Measurement/1 -> [Vab]
  Voltage Measurement1/1 -> [Vbc]
  Factor de Potencia/1 -> ϕ=acos(fdp)/1
  ϕ=acos(fdp)/1 -> Trigonometric Function/1
  Trigonometric Function/1 -> Potencia Reactiva=Potencia Activa*tan(ϕ)/2
  Potencia Reactiva=Potencia Activa*tan(ϕ)/1 -> Real-Imag to Complex1/2
  Cálculo potencia solar activa/1("Potencia solar activa ") -> Potencia Reactiva=Potencia Activa*tan(ϕ)/1, Real-Imag to Complex1/1
  Perfil de irradiancia/1 -> Cálculo potencia solar activa/1(Perfil de irradiancia)
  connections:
  Controlled Current Source1/LConn1 -- Controlled Current Source/LConn1 -- Ic/RConn1 -- Series RLC Branch1/RConn1 -- Voltage Measurement1/LConn2
  Controlled Current Source/RConn1 -- Voltage Measurement/LConn1 -- Ia/RConn1 -- Series RLC Branch/LConn1
  Series RLC Branch/RConn1 -- Ib/RConn1 -- Series RLC Branch1/LConn1 -- Voltage Measurement/LConn2 -- Voltage Measurement1/LConn1 -- Controlled Current Source1/RConn1

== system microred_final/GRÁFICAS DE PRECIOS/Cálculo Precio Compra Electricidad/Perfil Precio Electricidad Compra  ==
  note: Segundos-->Horas
  note: Tabla Precio Electricidad
  1-D Lookup Table : Lookup_n-D  NumberOfTableDimensions=1  BreakpointsForDimension1=Tiempo  Table=precioelectricidad_valores  InternalRulePriority=Speed  RndMeth=Simplest
  Clock : Clock
  Gain : Gain  Gain=1/(60*60)
  Precio compra : Scope
  Out2 : Outport  VectorParamsAs1DForOutWhenUnconnected=on
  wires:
  Gain/1 -> 1-D Lookup Table/1
  Clock/1 -> Gain/1
  1-D Lookup Table/1 -> Precio compra/1, Out2/1

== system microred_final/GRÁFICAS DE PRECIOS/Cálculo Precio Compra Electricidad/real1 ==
  In1 : Inport
  State Space : StateSpace  A=A  B=B  C=C  D=Dd  InitialCondition=X0
  Out1 : Outport  InitialOutput=0
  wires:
  In1/1 -> State Space/1
  State Space/1 -> Out1/1

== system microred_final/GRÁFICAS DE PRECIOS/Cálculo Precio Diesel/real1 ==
  In1 : Inport
  State Space : StateSpace  A=A  B=B  C=C  D=Dd  InitialCondition=X0
  Out1 : Outport  InitialOutput=0
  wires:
  In1/1 -> State Space/1
  State Space/1 -> Out1/1

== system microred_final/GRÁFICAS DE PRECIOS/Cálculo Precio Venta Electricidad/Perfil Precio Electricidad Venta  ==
  note: Tabla Precio Electricidad
  note: Segundos-->Horas
  1-D Lookup Table : Lookup_n-D  NumberOfTableDimensions=1  BreakpointsForDimension1=Tiempo  Table=Precioventaelectricidad  InternalRulePriority=Speed  RndMeth=Simplest
  Clock : Clock
  Gain : Gain  Gain=1/(60*60)
  Precio venta : Scope
  Out2 : Outport  VectorParamsAs1DForOutWhenUnconnected=on
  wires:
  Clock/1 -> Gain/1
  Gain/1 -> 1-D Lookup Table/1
  1-D Lookup Table/1 -> Precio venta/1, Out2/1

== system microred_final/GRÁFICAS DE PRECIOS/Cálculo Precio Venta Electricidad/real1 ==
  In1 : Inport
  State Space : StateSpace  A=A  B=B  C=C  D=Dd  InitialCondition=X0
  Out1 : Outport  InitialOutput=0
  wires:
  In1/1 -> State Space/1
  State Space/1 -> Out1/1

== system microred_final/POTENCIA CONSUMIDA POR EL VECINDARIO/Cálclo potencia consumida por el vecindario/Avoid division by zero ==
  I : Inport
  Complex to Magnitude-Angle : ComplexToMagnitudeAngle
  Magnitude-Angle to Complex : MagnitudeAngleToComplex
  Saturation1 : Saturate  UpperLimit=inf  LowerLimit=1e-6
  O : Outport
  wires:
  Complex to Magnitude-Angle/2 -> Magnitude-Angle to Complex/2
  Magnitude-Angle to Complex/1 -> O/1
  Complex to Magnitude-Angle/1 -> Saturation1/1
  Saturation1/1 -> Magnitude-Angle to Complex/1
  I/1 -> Complex to Magnitude-Angle/1

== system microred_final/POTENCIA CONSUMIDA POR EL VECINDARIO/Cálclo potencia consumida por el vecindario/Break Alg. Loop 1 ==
  In : Inport
  Complex to Real-Imag : ComplexToRealImag
  Real-Imag to Complex : RealImagToComplex
  imag : Subsystem  mask(Transfer Function with Initial Outputs){N=[1], D=[0.1  1], Y0=0, U0=0}
      mask prompts: N "Numerator:"; D "Denominator:"; Y0 "Initial output:"; U0 "Initial input:"
      mask help: Vector expressions for numerator, and denominator. Coefficients are in descending powers of s.
      mask init:
      | [A,B,C,Dd]=tf2ss(N,D);if (isempty(Y0));[m,n]=size(A);X0=zeros(1,m); end; if (isempty(U0));[m,p]=size(B);U0=zeros(1,p);end;X0=getxo(A,B,C,Dd,U0,Y0,0);
  real : Subsystem  mask(Transfer Function with Initial Outputs){N=[1], D=[0.1 1], Y0=0, U0=0}
      mask prompts: N "Numerator:"; D "Denominator:"; Y0 "Initial output:"; U0 "Initial input:"
      mask help: Vector expressions for numerator, and denominator. Coefficients are in descending powers of s.
      mask init:
      | [A,B,C,Dd]=tf2ss(N,D);if (isempty(Y0));[m,n]=size(A);X0=zeros(1,m); end; if (isempty(U0));[m,p]=size(B);U0=zeros(1,p);end;X0=getxo(A,B,C,Dd,U0,Y0,0);
  Out : Outport
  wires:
  Complex to Real-Imag/1 -> real/1(In1)
  Complex to Real-Imag/2 -> imag/1(In1)
  In/1 -> Complex to Real-Imag/1
  Real-Imag to Complex/1 -> Out/1
  real/1(Out1) -> Real-Imag to Complex/1
  imag/1(Out1) -> Real-Imag to Complex/2

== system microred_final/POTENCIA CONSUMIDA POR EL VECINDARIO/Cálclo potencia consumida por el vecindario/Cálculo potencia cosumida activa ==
  note: P(Activa)consumida=Perfil de consumo * Número de Casas
  Perfil de consumo : Inport
  Kw --> W : Gain  Gain=1000
  Número de casas : Gain  Gain=NumCasas
  a^1 : Gain  Gain=-1
  Potencia consumida activa : Outport
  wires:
  Perfil de consumo/1 -> Kw --> W/1
  Kw --> W/1 -> Número de casas/1
  Número de casas/1 -> a^1/1
  a^1/1 -> Potencia consumida activa/1

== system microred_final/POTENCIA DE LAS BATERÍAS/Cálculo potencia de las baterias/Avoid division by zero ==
  I : Inport
  Complex to Magnitude-Angle : ComplexToMagnitudeAngle
  Magnitude-Angle to Complex : MagnitudeAngleToComplex
  Saturation1 : Saturate  UpperLimit=inf  LowerLimit=1e-6
  O : Outport
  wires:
  Complex to Magnitude-Angle/2 -> Magnitude-Angle to Complex/2
  Magnitude-Angle to Complex/1 -> O/1
  Complex to Magnitude-Angle/1 -> Saturation1/1
  Saturation1/1 -> Magnitude-Angle to Complex/1
  I/1 -> Complex to Magnitude-Angle/1

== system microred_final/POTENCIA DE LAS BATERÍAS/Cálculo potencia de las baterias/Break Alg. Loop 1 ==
  In : Inport
  Complex to Real-Imag : ComplexToRealImag
  Real-Imag to Complex : RealImagToComplex
  imag : Subsystem  mask(Transfer Function with Initial Outputs){N=[1], D=[0.1  1], Y0=0, U0=0}
      mask prompts: N "Numerator:"; D "Denominator:"; Y0 "Initial output:"; U0 "Initial input:"
      mask help: Vector expressions for numerator, and denominator. Coefficients are in descending powers of s.
      mask init:
      | [A,B,C,Dd]=tf2ss(N,D);if (isempty(Y0));[m,n]=size(A);X0=zeros(1,m); end; if (isempty(U0));[m,p]=size(B);U0=zeros(1,p);end;X0=getxo(A,B,C,Dd,U0,Y0,0);
  real : Subsystem  mask(Transfer Function with Initial Outputs){N=[1], D=[0.1 1], Y0=0, U0=0}
      mask prompts: N "Numerator:"; D "Denominator:"; Y0 "Initial output:"; U0 "Initial input:"
      mask help: Vector expressions for numerator, and denominator. Coefficients are in descending powers of s.
      mask init:
      | [A,B,C,Dd]=tf2ss(N,D);if (isempty(Y0));[m,n]=size(A);X0=zeros(1,m); end; if (isempty(U0));[m,p]=size(B);U0=zeros(1,p);end;X0=getxo(A,B,C,Dd,U0,Y0,0);
  Out : Outport
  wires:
  Complex to Real-Imag/1 -> real/1(In1)
  Complex to Real-Imag/2 -> imag/1(In1)
  In/1 -> Complex to Real-Imag/1
  Real-Imag to Complex/1 -> Out/1
  real/1(Out1) -> Real-Imag to Complex/1
  imag/1(Out1) -> Real-Imag to Complex/2

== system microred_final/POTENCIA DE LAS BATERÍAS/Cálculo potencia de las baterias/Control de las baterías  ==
  Control de la potencia máxima : Subsystem
  Control del estado de carga (SOC) : Subsystem
  Cálculo del estado de carga (SOC) : Subsystem
  Potencia Baterias : Scope
  a^5 : Gain  Gain=-1
  Potencia Baterías : Outport
  SOC : Outport  Port=2
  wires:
  Cálculo del estado de carga (SOC)/1(SOC) -> SOC/1
  Control del estado de carga (SOC)/1(Potencia de las baterias) -> Potencia Baterias/1, a^5/1, [PotCargaDescarga], Cálculo del estado de carga (SOC)/1(Potencia de las baterias)
  Control de la potencia máxima/1("Potencia máxima ") -> Control del estado de carga (SOC)/1(Potencia máxima)
  a^5/1 -> Potencia Baterías/1

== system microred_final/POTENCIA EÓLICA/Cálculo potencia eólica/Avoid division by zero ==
  I : Inport
  Complex to Magnitude-Angle : ComplexToMagnitudeAngle
  Magnitude-Angle to Complex : MagnitudeAngleToComplex
  Saturation1 : Saturate  UpperLimit=inf  LowerLimit=1e-6
  O : Outport
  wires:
  Complex to Magnitude-Angle/2 -> Magnitude-Angle to Complex/2
  Magnitude-Angle to Complex/1 -> O/1
  Complex to Magnitude-Angle/1 -> Saturation1/1
  Saturation1/1 -> Magnitude-Angle to Complex/1
  I/1 -> Complex to Magnitude-Angle/1

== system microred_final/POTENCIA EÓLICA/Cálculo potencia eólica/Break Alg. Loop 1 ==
  In : Inport
  Complex to Real-Imag : ComplexToRealImag
  Real-Imag to Complex : RealImagToComplex
  imag : Subsystem  mask(Transfer Function with Initial Outputs){N=[1], D=[0.1  1], Y0=0, U0=0}
      mask prompts: N "Numerator:"; D "Denominator:"; Y0 "Initial output:"; U0 "Initial input:"
      mask help: Vector expressions for numerator, and denominator. Coefficients are in descending powers of s.
      mask init:
      | [A,B,C,Dd]=tf2ss(N,D);if (isempty(Y0));[m,n]=size(A);X0=zeros(1,m); end; if (isempty(U0));[m,p]=size(B);U0=zeros(1,p);end;X0=getxo(A,B,C,Dd,U0,Y0,0);
  real : Subsystem  mask(Transfer Function with Initial Outputs){N=[1], D=[0.1 1], Y0=0, U0=0}
      mask prompts: N "Numerator:"; D "Denominator:"; Y0 "Initial output:"; U0 "Initial input:"
      mask help: Vector expressions for numerator, and denominator. Coefficients are in descending powers of s.
      mask init:
      | [A,B,C,Dd]=tf2ss(N,D);if (isempty(Y0));[m,n]=size(A);X0=zeros(1,m); end; if (isempty(U0));[m,p]=size(B);U0=zeros(1,p);end;X0=getxo(A,B,C,Dd,U0,Y0,0);
  Out : Outport
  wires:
  Complex to Real-Imag/1 -> real/1(In1)
  Complex to Real-Imag/2 -> imag/1(In1)
  In/1 -> Complex to Real-Imag/1
  Real-Imag to Complex/1 -> Out/1
  real/1(Out1) -> Real-Imag to Complex/1
  imag/1(Out1) -> Real-Imag to Complex/2
